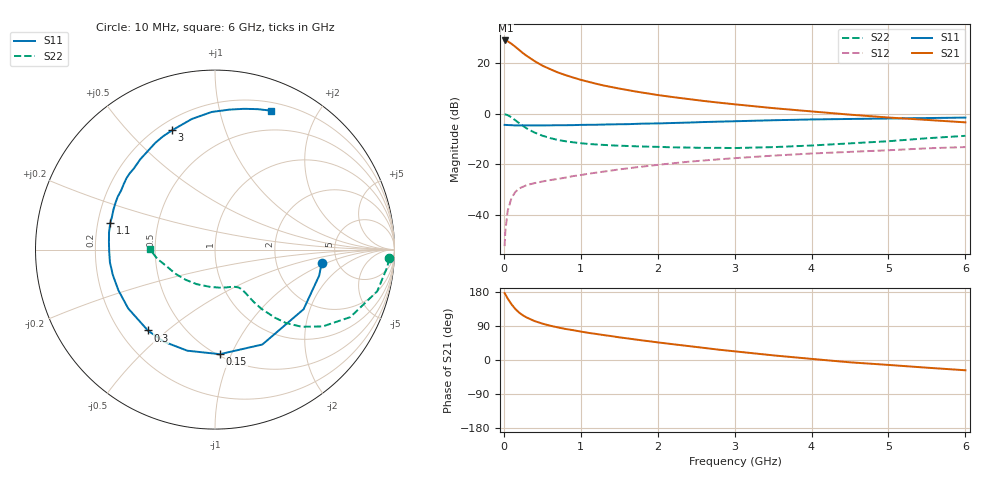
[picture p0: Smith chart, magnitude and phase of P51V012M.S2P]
! SIEMENS Small Signal Semiconductors
! BFP183
! Si NPN RF Bipolar Junction Transistor in SOT143
! VCE = 1 V  IC = 12 mA
! Common Emitter S-Parameters:  March  1996
# GHz  S  MA  R  50
!  f  S11  S21  S12  S22
! GHz  MAG  ANG  MAG  ANG  MAG  ANG  MAG  ANG
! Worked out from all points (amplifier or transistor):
!   36 points, 10 MHz to 6 GHz, reference 50 ohm
!   highest |S21| = 28.9 dB at 20 MHz (marker M1)
!   |S21| within 3 dB of that: start of sweep to 169.6 MHz
!   unconditionally stable (mu >= 1): 921.9 MHz to end of sweep
!   at 250 MHz: K = 0.39, MSG = 26.4 dB, |S12| = -28.9 dB
!   at 1.4 GHz: K = 1.16, MAG = 14.1 dB, |S12| = -22.5 dB
!   at 6 GHz: K = 1.01, MAG = 4.3 dB, |S12| = -13.2 dB
!   S11 on the Smith chart (normalised r, x): 10 MHz: 3.77, -0.87; 150 MHz: 0.51, -0.91; 300 MHz: 0.31, -0.43; 1.1 GHz: 0.25, +0.12; 3 GHz: 0.25, +0.67; 6 GHz: 0.28, +1.44
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0.01  0.5989 -7.1  27.84 176.5  0.0024 84.7  0.9725 -2.9
0.02  0.5984 -14.0  27.93 173.1  0.0048 76.2  0.9645 -5.8
0.05  0.595 -34.0  26.95 162.2  0.012 78.3  0.9331 -14.4
0.1  0.5909 -63.5  23.97 146.9  0.0216 62.7  0.8426 -26.5
0.15  0.5833 -87.3  20.93 134.5  0.0284 55.6  0.7372 -35.5
0.2  0.584 -105.3  18.1 124.9  0.0332 49.5  0.6461 -41.7
0.25  0.5867 -119.0  15.64 117.5  0.0359 45.6  0.5703 -45.9
0.3  0.5857 -129.7  13.77 111.8  0.0388 43.1  0.5065 -48.6
0.4  0.5843 -145.9  10.89 102.7  0.0423 41.7  0.4216 -51.8
0.5  0.584 -157.2  8.901 96.1  0.0455 40.4  0.367 -53.4
0.6  0.5867 -166.1  7.595 90.6  0.0485 40.8  0.329 -54.2
0.7  0.5897 -173.2  6.531 86.1  0.0512 41.7  0.3026 -54.7
0.8  0.5897 -179.3  5.785 82.0  0.0543 42.3  0.2845 -55.3
1.1  0.6019 165.9  4.253 71.6  0.0649 44.1  0.2518 -57.7
1.5  0.6169 151.4  3.129 59.8  0.079 44.8  0.2321 -63.0
1.8  0.6336 141.1  2.605 51.7  0.0897 44.3  0.224 -68.7
2.2  0.6531 129.6  2.12 41.6  0.1044 42.4  0.2157 -78.1
3  0.7063 109.8  1.528 22.9  0.1317 36.8  0.2089 -101.5
3.5  0.7393 100.0  1.284 12.3  0.1478 33.1  0.2176 -117.6
4.5  0.7839 84.2  0.954 -6.1  0.1754 24.6  0.2583 -148.7
5.5  0.8174 73.2  0.751 -20.3  0.2061 17.2  0.3258 -171.0
6  0.835 68.0  0.672 -27.1  0.2182 12.5  0.3641 179.5
